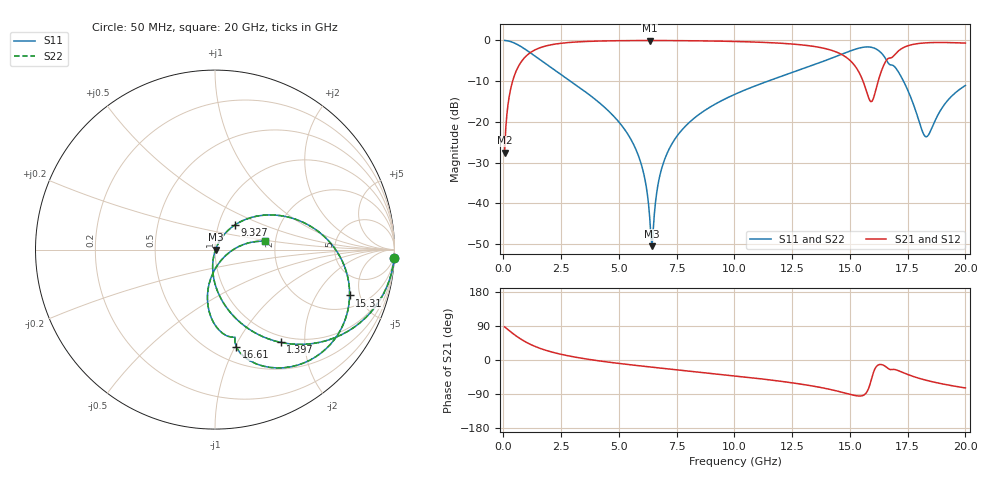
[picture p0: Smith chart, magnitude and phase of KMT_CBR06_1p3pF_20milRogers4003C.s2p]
! Data measured by Modelithics Inc. support@modelithics.com 813-866-6335
! KEMET CBR0603 1.3pF, Pad Width= 0.851mm, Pad Length= 0.64mm, Pad Gap= 0.62mm, 20mil Rogers 4003C substrate Data, January 2022
# hz S ma R 50
! 2 Port Network Data from SP1.SP block
! freq  magS11  angS11  magS21  angS21  magS12  angS12  magS22  angS22
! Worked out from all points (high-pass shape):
!   401 points, 50 MHz to 20 GHz, reference 50 ohm
!   highest |S21| = -0.03 dB at 6.334 GHz (marker M1); lowest = -27.6 dB at 50 MHz (marker M2)
!   |S21| within 3 dB of the highest: 1.157 GHz to 14.49 GHz (13.33 GHz wide, 170 % of centre); 17.02 GHz to end of sweep
!   lowest |S11| = -50.5 dB at 6.434 GHz (marker M3), VSWR 1.01, Z = 50.3 - j0.0509 ohm
!   |S11| at or under -10 dB: 2.903 GHz to 11.45 GHz (8.546 GHz wide, 119 % of centre); 17.32 GHz to end of sweep
!   |S22| runs from -50.5 to 0.0 dB; largest |S21 - S12| = 0
!   S11 on the Smith chart (normalised r, x): 50 MHz: 1, -45; 1.397 GHz: 0.90, -1.54; 9.327 GHz: 1.19, +0.34; 15.31 GHz: 2.91, -4.00; 16.61 GHz: 0.64, -1.01; 20 GHz: 1.75, +0.18
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5e7  0.9991 -2.5  0.04182 87.4  0.04182 87.4  0.9991 -2.5
2.495e8  0.9787 -12.6  0.2047 77.4  0.2047 77.4  0.9787 -12.6
4.49e8  0.9353 -22.0  0.3531 67.9  0.3531 67.9  0.9353 -22.0
1.396625e9  0.6327 -54.7  0.7728 35.1  0.7728 35.1  0.6327 -54.7
3.391625e9  0.2521 -84.9  0.9654 4.6  0.9654 4.6  0.2521 -84.9
5.586125e9  0.05617 -100.5  0.9955 -13.3  0.9955 -13.3  0.05617 -100.5
6.084875e9  0.02234 -99.3  0.9967 -16.7  0.9967 -16.7  0.02234 -99.3
6.33425e9  0.00659 -82.1  0.9968 -18.3  0.9968 -18.3  0.00659 -82.1
6.434e9  0.002974 -9.8  0.9968 -19.0  0.9968 -19.0  0.002974 -9.8
6.73325e9  0.01954 60.2  0.9966 -20.9  0.9966 -20.9  0.01954 60.2
7.581125e9  0.07087 61.0  0.9939 -26.3  0.9939 -26.3  0.07087 61.0
9.32675e9  0.1748 51.2  0.9801 -37.4  0.9801 -37.4  0.1748 51.2
1.0025e10  0.2183 46.8  0.9708 -42.0  0.9708 -42.0  0.2183 46.8
1.336662e10  0.4931 19.3  0.8503 -68.5  0.8503 -68.5  0.4931 19.3
1.451375e10  0.6546 2.1  0.7005 -82.9  0.7005 -82.9  0.6546 2.1
1.531175e10  0.7923 -18.8  0.4457 -94.7  0.4457 -94.7  0.7923 -18.8
1.591025e10  0.8257 -44.1  0.1766 -55.6  0.1766 -55.6  0.8257 -44.1
1.66085e10  0.5565 -77.6  0.5837 -20.1  0.5837 -20.1  0.5565 -77.6
1.670825e10  0.5079 -77.4  0.6075 -24.5  0.6075 -24.5  0.5079 -77.4
1.735662e10  0.3012 -97.8  0.8265 -34.6  0.8265 -34.6  0.3012 -97.8
1.830425e10  0.06544 -43.6  0.9348 -53.5  0.9348 -53.5  0.06544 -43.6
2e10  0.2799 9.5  0.927 -73.8  0.927 -73.8  0.2799 9.5
